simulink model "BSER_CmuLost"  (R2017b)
settings: Solver=FixedStepDiscrete  StartTime=0.0  StopTime=10.0  FixedStep=0.02  RelTol=1e-3  EnableMultiTasking=on
undefined symbols (not defined in the file or in its folder): BSER_tiBattChrgCmuLost_C, BSER_tiBattDisChrgCmuLost_C
libraries: simulink x12

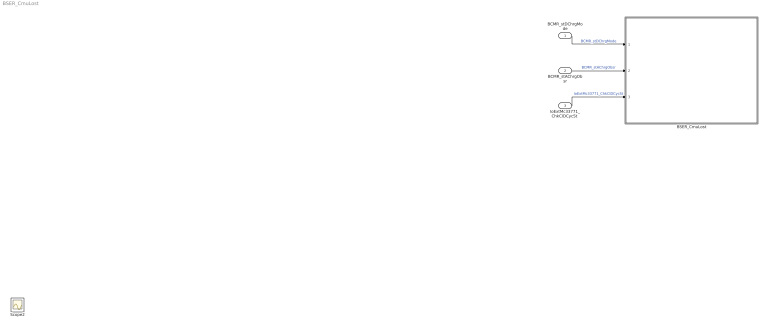
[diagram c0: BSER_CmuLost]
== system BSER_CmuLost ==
  BCMR_stDChrgMode : Inport
  BCMR_stAChrgObsr : Inport  Port=2
  "IoExtMc33771_ChkCIDCycSt " : Inport  Port=3
  BSER_CmuLost : Subsystem
  Scope2 : Scope
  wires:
  BCMR_stDChrgMode/1 -> BSER_CmuLost/1(BCMR_stDChrgMode)  "BCMR_stDChrgMode"
  BCMR_stAChrgObsr/1 -> BSER_CmuLost/2(BCMR_stAChrgObsr)  "BCMR_stAChrgObsr"
  "IoExtMc33771_ChkCIDCycSt "/1 -> BSER_CmuLost/3("IoExtMc33771_ChkCIDCycSt ")  "IoExtMc33771_ChkCIDCycSt"

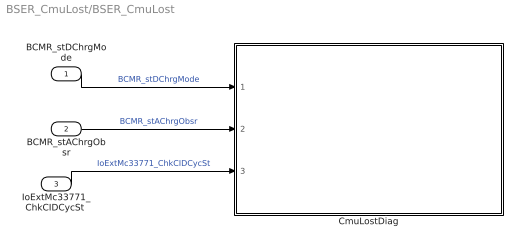
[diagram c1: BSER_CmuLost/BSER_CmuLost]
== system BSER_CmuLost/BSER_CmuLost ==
  BCMR_stDChrgMode : Inport
  BCMR_stAChrgObsr : Inport  Port=2
  "IoExtMc33771_ChkCIDCycSt " : Inport  Port=3
  CmuLostDiag : Subsystem
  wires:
  BCMR_stDChrgMode/1 -> CmuLostDiag/1(BCMR_stDChrgMode)  "BCMR_stDChrgMode"
  BCMR_stAChrgObsr/1 -> CmuLostDiag/2(BCMR_stAChrgObsr)  "BCMR_stAChrgObsr"
  "IoExtMc33771_ChkCIDCycSt "/1 -> CmuLostDiag/3("IoExtMc33771_ChkCIDCycSt ")  "IoExtMc33771_ChkCIDCycSt"

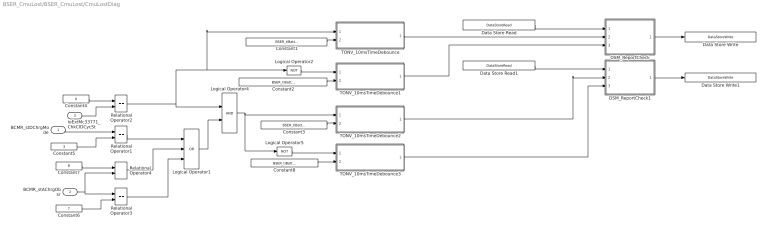
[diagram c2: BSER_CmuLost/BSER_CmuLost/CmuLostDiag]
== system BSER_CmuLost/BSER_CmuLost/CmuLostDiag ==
  BCMR_stDChrgMode : Inport
  BCMR_stAChrgObsr : Inport  Port=2
  "IoExtMc33771_ChkCIDCycSt " : Inport  Port=3
  Constant1 : Constant  Value=BSER_tiBattDisChrgCmuLost_C
  Constant2 : Constant  Value=BSER_tiBattDisChrgCmuLost_C
  Constant3 : Constant  Value=BSER_tiBattChrgCmuLost_C
  Constant4 : Constant  Value=0  OutDataTypeStr=uint8
  Constant5 : Constant  Value=3  OutDataTypeStr=uint8
  Constant6 : Constant  Value=7  OutDataTypeStr=uint8
  Constant7 : Constant  Value=8  OutDataTypeStr=uint8
  Constant8 : Constant  Value=BSER_tiBattChrgCmuLost_C
  DSM_ReportCheck : Subsystem  TreatAsAtomicUnit=on  RTWFcnName=DSM_ReportCheck  RTWFileName=SrvLib
  DSM_ReportCheck1 : Subsystem  TreatAsAtomicUnit=on  RTWFcnName=DSM_ReportCheck  RTWFileName=SrvLib
  Data Store Read : DataStoreRead  DataStoreName=DFC_DisChrgCmuLost
  Data Store Read1 : DataStoreRead  DataStoreName=DFC_ChrgCmuLost
  Data Store Write : DataStoreWrite  DataStoreName=DFC_DisChrgCmuLost
  Data Store Write1 : DataStoreWrite  DataStoreName=DFC_ChrgCmuLost
  Logical Operator1 : Logic  Operator=OR  Inputs=3  AllPortsSameDT=off  OutDataTypeStr=boolean
  Logical Operator2 : Logic  Operator=NOT  AllPortsSameDT=off  OutDataTypeStr=boolean
  Logical Operator4 : Logic  AllPortsSameDT=off  OutDataTypeStr=boolean
  Logical Operator5 : Logic  Operator=NOT  AllPortsSameDT=off  OutDataTypeStr=boolean
  Relational Operator{1..4} (4 alike) : RelationalOperator  Operator===  OutDataTypeStr=boolean  RndMeth=Simplest
  TONV_10msTimeDebounce : Subsystem  TreatAsAtomicUnit=on  RTWFcnName=TONV_10msTimeDebounce  RTWFileName=SrvLib
  TONV_10msTimeDebounce1 : Subsystem  TreatAsAtomicUnit=on  RTWFcnName=TONV_10msTimeDebounce  RTWFileName=SrvLib
  TONV_10msTimeDebounce2 : Subsystem  TreatAsAtomicUnit=on  RTWFcnName=TONV_10msTimeDebounce  RTWFileName=SrvLib
  TONV_10msTimeDebounce3 : Subsystem  TreatAsAtomicUnit=on  RTWFcnName=TONV_10msTimeDebounce  RTWFileName=SrvLib
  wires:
  Constant1/1 -> TONV_10msTimeDebounce/2(T)
  Relational Operator2/1 -> Logical Operator2/1, TONV_10msTimeDebounce/1(u), Logical Operator4/1
  Constant2/1 -> TONV_10msTimeDebounce1/2(T)
  Logical Operator2/1 -> TONV_10msTimeDebounce1/1(u)
  TONV_10msTimeDebounce/1(y) -> DSM_ReportCheck/2(Err)
  TONV_10msTimeDebounce1/1(y) -> DSM_ReportCheck/3(Heal)
  TONV_10msTimeDebounce3/1(y) -> DSM_ReportCheck1/3(Heal)
  TONV_10msTimeDebounce2/1(y) -> DSM_ReportCheck1/2(Err)
  Constant3/1 -> TONV_10msTimeDebounce2/2(T)
  Constant4/1 -> Relational Operator2/1
  "IoExtMc33771_ChkCIDCycSt "/1 -> Relational Operator2/2
  BCMR_stDChrgMode/1 -> Relational Operator1/1
  Constant5/1 -> Relational Operator1/2
  BCMR_stAChrgObsr/1 -> Relational Operator4/2, Relational Operator3/1
  Constant6/1 -> Relational Operator3/2
  Constant7/1 -> Relational Operator4/1
  Relational Operator1/1 -> Logical Operator1/1
  Relational Operator4/1 -> Logical Operator1/2
  Relational Operator3/1 -> Logical Operator1/3
  Logical Operator1/1 -> Logical Operator4/2
  Logical Operator4/1 -> Logical Operator5/1, TONV_10msTimeDebounce2/1(u)
  Logical Operator5/1 -> TONV_10msTimeDebounce3/1(u)
  Constant8/1 -> TONV_10msTimeDebounce3/2(T)
  Data Store Read/1 -> DSM_ReportCheck/1(Dfc_id_nv)
  DSM_ReportCheck/1(Dfc_id) -> Data Store Write/1
  Data Store Read1/1 -> DSM_ReportCheck1/1(Dfc_id_nv)
  DSM_ReportCheck1/1(Dfc_id) -> Data Store Write1/1

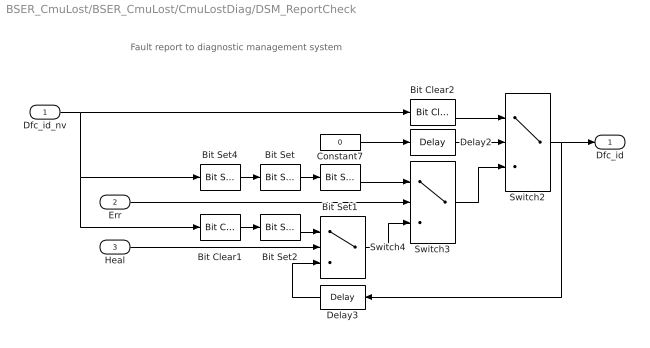
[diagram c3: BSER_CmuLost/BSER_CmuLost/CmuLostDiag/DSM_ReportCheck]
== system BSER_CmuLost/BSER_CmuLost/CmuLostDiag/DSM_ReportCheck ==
  note: Fault report to diagnostic management system
  Dfc_id_nv : Inport  OutDataTypeStr=uint8
  Err : Inport  Port=2
  Heal : Inport  Port=3
  Bit Clear1 : simulink/Logic and Bit Operations/Bit Clear  iBit=4
  Bit Clear2 : simulink/Logic and Bit Operations/Bit Clear  iBit=3
  Bit Set : simulink/Logic and Bit Operations/Bit Set  iBit=4
  Bit Set1 : simulink/Logic and Bit Operations/Bit Set  iBit=3
  Bit Set2 : simulink/Logic and Bit Operations/Bit Set  iBit=3
  Bit Set4 : simulink/Logic and Bit Operations/Bit Set  iBit=7
  Constant7 : Constant  Value=0  OutDataTypeStr=boolean
  Delay2 : Delay  DelayLength=1  InitialCondition=1
  Delay3 : Delay  DelayLength=1  InitialCondition=0
  Switch2 : Switch  Criteria=u2 ~= 0
  Switch3 : Switch  Criteria=u2 ~= 0
  Switch4 : Switch  Criteria=u2 ~= 0
  Dfc_id : Outport  OutDataTypeStr=uint8
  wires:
  Dfc_id_nv/1 -> Bit Clear2/1, Bit Set4/1, Bit Clear1/1
  Bit Set4/1 -> Bit Set/1
  Constant7/1 -> Delay2/1
  Delay2/1 -> Switch2/2
  Switch3/1 -> Switch2/3
  Bit Clear2/1 -> Switch2/1
  Switch2/1 -> Delay3/1, Dfc_id/1
  Bit Set1/1 -> Switch3/1
  Bit Set/1 -> Bit Set1/1
  Switch4/1 -> Switch3/3
  Err/1 -> Switch3/2
  Bit Set2/1 -> Switch4/1
  Bit Clear1/1 -> Bit Set2/1
  Delay3/1 -> Switch4/3
  Heal/1 -> Switch4/2

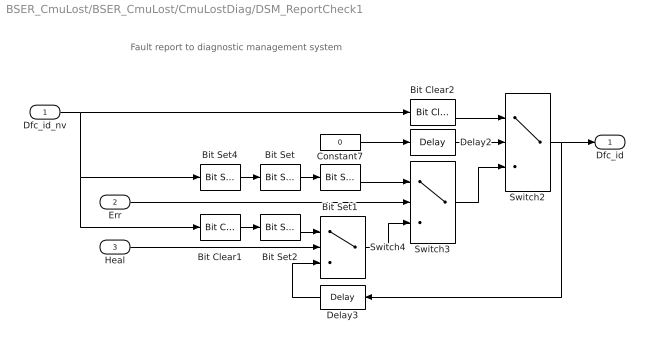
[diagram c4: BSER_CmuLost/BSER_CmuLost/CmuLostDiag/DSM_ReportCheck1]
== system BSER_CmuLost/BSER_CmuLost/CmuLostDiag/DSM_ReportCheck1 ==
  note: Fault report to diagnostic management system
  Dfc_id_nv : Inport  OutDataTypeStr=uint8
  Err : Inport  Port=2
  Heal : Inport  Port=3
  Bit Clear1 : simulink/Logic and Bit Operations/Bit Clear  iBit=4
  Bit Clear2 : simulink/Logic and Bit Operations/Bit Clear  iBit=3
  Bit Set : simulink/Logic and Bit Operations/Bit Set  iBit=4
  Bit Set1 : simulink/Logic and Bit Operations/Bit Set  iBit=3
  Bit Set2 : simulink/Logic and Bit Operations/Bit Set  iBit=3
  Bit Set4 : simulink/Logic and Bit Operations/Bit Set  iBit=7
  Constant7 : Constant  Value=0  OutDataTypeStr=boolean
  Delay2 : Delay  DelayLength=1  InitialCondition=1
  Delay3 : Delay  DelayLength=1  InitialCondition=0
  Switch2 : Switch  Criteria=u2 ~= 0
  Switch3 : Switch  Criteria=u2 ~= 0
  Switch4 : Switch  Criteria=u2 ~= 0
  Dfc_id : Outport  OutDataTypeStr=uint8
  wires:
  Heal/1 -> Switch4/2
  Delay3/1 -> Switch4/3
  Bit Clear1/1 -> Bit Set2/1
  Bit Set2/1 -> Switch4/1
  Err/1 -> Switch3/2
  Switch4/1 -> Switch3/3
  Bit Set/1 -> Bit Set1/1
  Bit Set1/1 -> Switch3/1
  Switch2/1 -> Dfc_id/1, Delay3/1
  Bit Clear2/1 -> Switch2/1
  Switch3/1 -> Switch2/3
  Delay2/1 -> Switch2/2
  Constant7/1 -> Delay2/1
  Bit Set4/1 -> Bit Set/1
  Dfc_id_nv/1 -> Bit Clear1/1, Bit Set4/1, Bit Clear2/1

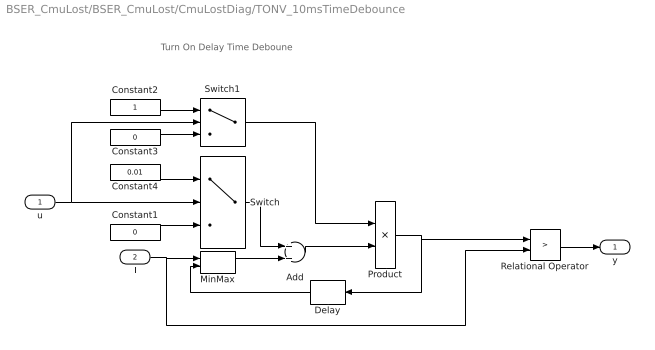
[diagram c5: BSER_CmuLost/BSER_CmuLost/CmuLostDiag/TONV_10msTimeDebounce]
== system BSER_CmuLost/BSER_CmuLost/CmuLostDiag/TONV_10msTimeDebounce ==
  note: Turn On Delay Time Deboune
  u : Inport
  T : Inport  Port=2
  Add : Sum
  Constant1 : Constant  Value=0  OutDataTypeStr=single
  Constant2 : Constant  OutDataTypeStr=uint8
  Constant3 : Constant  Value=0  OutDataTypeStr=uint8
  Constant4 : Constant  Value=0.01  OutDataTypeStr=single
  Delay : Delay  DelayLength=1  InitialCondition=0
  MinMax : MinMax  Inputs=2
  Product : Product  OutMin=[0]  OutMax=[65535]  OutDataTypeStr=single
  Relational Operator : RelationalOperator  Operator=>  OutDataTypeStr=boolean  RndMeth=Simplest
  Switch : Switch  Criteria=u2 ~= 0
  Switch1 : Switch  Criteria=u2 ~= 0
  y : Outport
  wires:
  MinMax/1 -> Add/2
  T/1 -> Relational Operator/2, MinMax/1
  Relational Operator/1 -> y/1
  Delay/1 -> MinMax/2
  Switch/1 -> Add/1
  Product/1 -> Delay/1, Relational Operator/1
  Add/1 -> Product/2
  Constant1/1 -> Switch/3
  Constant4/1 -> Switch/1
  u/1 -> Switch/2, Switch1/2
  Constant2/1 -> Switch1/1
  Constant3/1 -> Switch1/3
  Switch1/1 -> Product/1

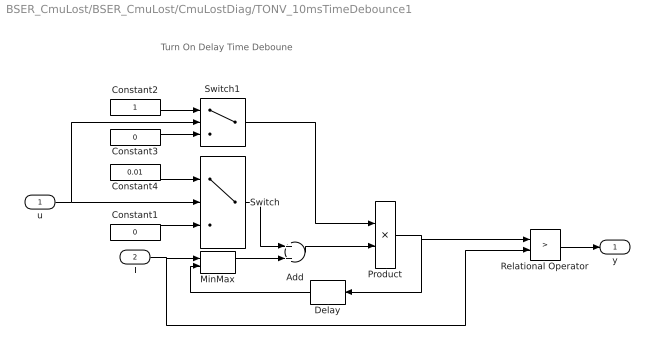
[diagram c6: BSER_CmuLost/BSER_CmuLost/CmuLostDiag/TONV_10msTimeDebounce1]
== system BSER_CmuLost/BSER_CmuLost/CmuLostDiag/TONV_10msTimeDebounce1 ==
  note: Turn On Delay Time Deboune
  u : Inport
  T : Inport  Port=2
  Add : Sum
  Constant1 : Constant  Value=0  OutDataTypeStr=single
  Constant2 : Constant  OutDataTypeStr=uint8
  Constant3 : Constant  Value=0  OutDataTypeStr=uint8
  Constant4 : Constant  Value=0.01  OutDataTypeStr=single
  Delay : Delay  DelayLength=1  InitialCondition=0
  MinMax : MinMax  Inputs=2
  Product : Product  OutMin=[0]  OutMax=[65535]  OutDataTypeStr=single
  Relational Operator : RelationalOperator  Operator=>  OutDataTypeStr=boolean  RndMeth=Simplest
  Switch : Switch  Criteria=u2 ~= 0
  Switch1 : Switch  Criteria=u2 ~= 0
  y : Outport
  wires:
  Switch1/1 -> Product/1
  Constant3/1 -> Switch1/3
  Constant2/1 -> Switch1/1
  u/1 -> Switch1/2, Switch/2
  Constant4/1 -> Switch/1
  Constant1/1 -> Switch/3
  Add/1 -> Product/2
  Product/1 -> Relational Operator/1, Delay/1
  Switch/1 -> Add/1
  Delay/1 -> MinMax/2
  Relational Operator/1 -> y/1
  T/1 -> MinMax/1, Relational Operator/2
  MinMax/1 -> Add/2

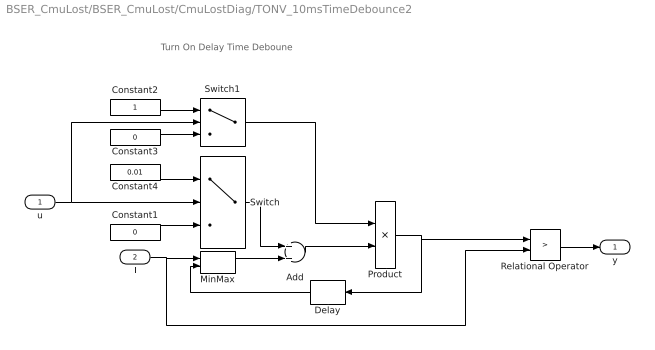
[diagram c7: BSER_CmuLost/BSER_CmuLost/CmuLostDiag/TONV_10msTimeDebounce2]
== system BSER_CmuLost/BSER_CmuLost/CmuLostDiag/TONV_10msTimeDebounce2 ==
  note: Turn On Delay Time Deboune
  u : Inport
  T : Inport  Port=2
  Add : Sum
  Constant1 : Constant  Value=0  OutDataTypeStr=single
  Constant2 : Constant  OutDataTypeStr=uint8
  Constant3 : Constant  Value=0  OutDataTypeStr=uint8
  Constant4 : Constant  Value=0.01  OutDataTypeStr=single
  Delay : Delay  DelayLength=1  InitialCondition=0
  MinMax : MinMax  Inputs=2
  Product : Product  OutMin=[0]  OutMax=[65535]  OutDataTypeStr=single
  Relational Operator : RelationalOperator  Operator=>  OutDataTypeStr=boolean  RndMeth=Simplest
  Switch : Switch  Criteria=u2 ~= 0
  Switch1 : Switch  Criteria=u2 ~= 0
  y : Outport
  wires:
  MinMax/1 -> Add/2
  T/1 -> Relational Operator/2, MinMax/1
  Relational Operator/1 -> y/1
  Delay/1 -> MinMax/2
  Switch/1 -> Add/1
  Product/1 -> Delay/1, Relational Operator/1
  Add/1 -> Product/2
  Constant1/1 -> Switch/3
  Constant4/1 -> Switch/1
  u/1 -> Switch/2, Switch1/2
  Constant2/1 -> Switch1/1
  Constant3/1 -> Switch1/3
  Switch1/1 -> Product/1

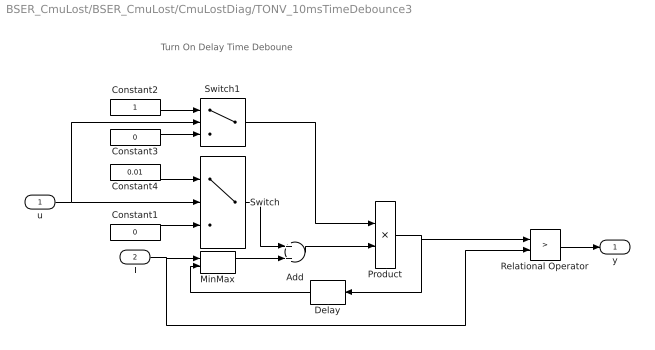
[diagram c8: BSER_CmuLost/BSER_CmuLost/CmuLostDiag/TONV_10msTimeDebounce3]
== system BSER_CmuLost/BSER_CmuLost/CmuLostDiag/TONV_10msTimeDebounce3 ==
  note: Turn On Delay Time Deboune
  u : Inport
  T : Inport  Port=2
  Add : Sum
  Constant1 : Constant  Value=0  OutDataTypeStr=single
  Constant2 : Constant  OutDataTypeStr=uint8
  Constant3 : Constant  Value=0  OutDataTypeStr=uint8
  Constant4 : Constant  Value=0.01  OutDataTypeStr=single
  Delay : Delay  DelayLength=1  InitialCondition=0
  MinMax : MinMax  Inputs=2
  Product : Product  OutMin=[0]  OutMax=[65535]  OutDataTypeStr=single
  Relational Operator : RelationalOperator  Operator=>  OutDataTypeStr=boolean  RndMeth=Simplest
  Switch : Switch  Criteria=u2 ~= 0
  Switch1 : Switch  Criteria=u2 ~= 0
  y : Outport
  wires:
  Switch1/1 -> Product/1
  Constant3/1 -> Switch1/3
  Constant2/1 -> Switch1/1
  u/1 -> Switch1/2, Switch/2
  Constant4/1 -> Switch/1
  Constant1/1 -> Switch/3
  Add/1 -> Product/2
  Product/1 -> Relational Operator/1, Delay/1
  Switch/1 -> Add/1
  Delay/1 -> MinMax/2
  Relational Operator/1 -> y/1
  T/1 -> MinMax/1, Relational Operator/2
  MinMax/1 -> Add/2
